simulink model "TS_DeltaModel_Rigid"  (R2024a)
settings: Solver=ode45  StartTime=0  StopTime=2  FixedStep=1e-4  EnableMultiTasking=on
PreLoadFcn:
  | warning('off','sm:sli:setup:compile:LocalSolverNotSupported')
InitFcn:
  |  SimParam.IC = SM2_InitCondConstrFnc(RawParam,IC);
model workspace (MAT data in the model file):
  op_trim1 : opcond.OperatingReport (value not decoded)
  op_trim3 : opcond.OperatingReport (value not decoded)
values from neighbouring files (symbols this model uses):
  RawParam = RobotParamGather(ParamLib)    [DeltaModelMain_v2.m]    (also in main_TimeSimulation.m; MGI.m = y)
libraries: SM2_BallJointPartsLib x6, SM2_ForeArmPartsLib x6, simulink x6, SM2_ArmPartsLib x3, SM2_MotorPartsLib x3, SM2_FramePartsLib x1, ElecDriverLib x1, SM2_ToolPartsLib x1

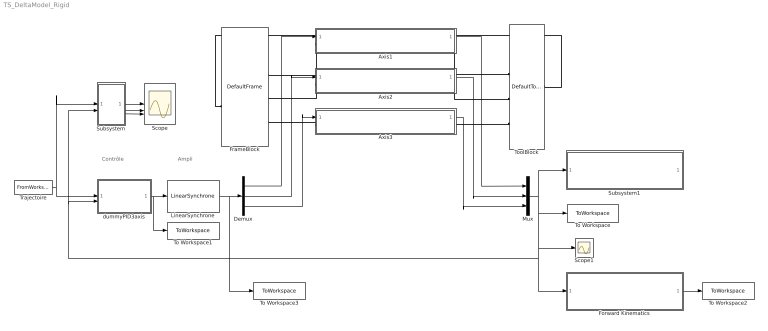
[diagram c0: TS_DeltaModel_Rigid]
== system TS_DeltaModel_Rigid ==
  note: Contrôle
  note: Ampli
  Axis1 : Subsystem  mask{AxisID=1}
      mask prompts: AxisID "Axis ID number (1,2 or 3)"
  Axis2 : Subsystem  mask{AxisID=2}
      mask prompts: AxisID "Axis ID number (1,2 or 3)"
  Axis3 : Subsystem  mask{AxisID=3}
      mask prompts: AxisID "Axis ID number (1,2 or 3)"
  Demux : Demux  Outputs=3
  Forward Kinematics : Subsystem
  FrameBlock : SM2_FramePartsLib/DefaultFrame  SystemSampleTime=-1  VariantActivationTime=update diagram  AllowFlexibleInterface=on  Latency=0  AutoFrameSizeCalculation=off
  LinearSynchrone : ElecDriverLib/LinearSynchrone  SystemSampleTime=-1  VariantControl=driverVarLinearSynchrone  VariantActivationTime=update diagram  AllowFlexibleInterface=on  Latency=0  AutoFrameSizeCalculation=off
  Mux : Mux  Inputs=3
  Scope : Scope  NumInputPorts=3
  Scope1 : Scope
  Subsystem : Subsystem
  Subsystem1 : Subsystem
  To Workspace : ToWorkspace  VariableName=angleData  SaveFormat=Timeseries  SampleTime=-1
  To Workspace1 : ToWorkspace  VariableName=controlData  SaveFormat=Timeseries  SampleTime=-1
  To Workspace2 : ToWorkspace  VariableName=endEffectorPos  SaveFormat=Structure With Time  SampleTime=-1
  To Workspace3 : ToWorkspace  VariableName=Torques  SaveFormat=Structure With Time  SampleTime=-1
  ToolBlock : SM2_ToolPartsLib/DefaultTool  SystemSampleTime=-1  VariantActivationTime=update diagram  AllowFlexibleInterface=on  Latency=0  AutoFrameSizeCalculation=off
      link override NacelleGraph: ExtrusionLength=0.005  Mass=SimParam.Tool.m
  Trajectoire : FromWorkspace  VariableName=simin  SampleTime=SimParam.Control.Te  ZeroCross=off  OutputAfterFinalValue=Holding final value
  dummyPID3axis : Subsystem  InitFcn=SimParam.Control = Control_ParamInitFnc(RawParam,3);  VariantControl=controlVarDefault
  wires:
  LinearSynchrone/1 -> To Workspace3/1, Demux/1
  Mux/1 -> Scope1/1, Forward Kinematics/1(q), Subsystem/2(y), dummyPID3axis/2(Alpha), To Workspace/1, Subsystem1/1(In1)
  dummyPID3axis/1(U) -> To Workspace1/1, LinearSynchrone/1
  Trajectoire/1 -> Subsystem/1(y_c), dummyPID3axis/1(Alpha_c)
  Demux/2 -> Axis2/1(Torque)
  Demux/3 -> Axis3/1(Torque)
  Axis1/1(Alpha) -> Mux/1
  Axis2/1(Alpha) -> Mux/2
  Axis3/1(Alpha) -> Mux/3
  Demux/1 -> Axis1/1(Torque)
  Subsystem/1(axe1) -> Scope/1
  Subsystem/2(axe2) -> Scope/2
  Subsystem/3(axe3) -> Scope/3
  Forward Kinematics/1(Out1) -> To Workspace2/1
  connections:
  Axis1/LConn1 -- FrameBlock/RConn1
  Axis2/LConn1 -- FrameBlock/RConn2
  Axis3/LConn1 -- FrameBlock/RConn3
  Axis3/RConn1 -- ToolBlock/RConn3
  Axis2/RConn1 -- ToolBlock/RConn2
  Axis1/RConn1 -- ToolBlock/RConn1
  FrameBlock/LConn1 -- ToolBlock/LConn1

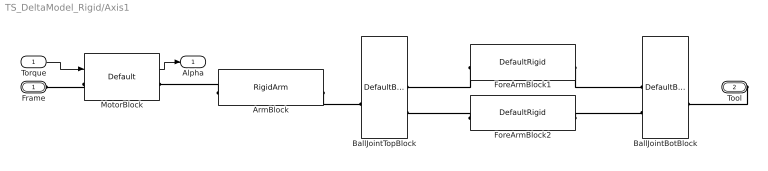
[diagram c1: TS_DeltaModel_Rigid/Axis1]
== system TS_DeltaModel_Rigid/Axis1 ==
  Torque : Inport
  ArmBlock : SM2_ArmPartsLib/RigidArm  SystemSampleTime=-1  VariantControl=armVarDefault  VariantActivationTime=update diagram  AllowFlexibleInterface=on  Latency=0  AutoFrameSizeCalculation=off
      link override ArmGraph: ExtrusionCrossSection=[5.5e-3 0; 2.75e-3 4.76e-3; -2.75e-3 4.76e-3; -5.5e-3 0; -2.75e-3 -4.76e-3; 2.75e-3 -4.76e-3; 5.5e-3 0]
  BallJointBotBlock : SM2_BallJointPartsLib/DefaultBallJointBotPair  SystemSampleTime=-1  VariantActivationTime=update diagram  AllowFlexibleInterface=on  Latency=0  AutoFrameSizeCalculation=off
  BallJointTopBlock : SM2_BallJointPartsLib/DefaultBallJointTopPair  SystemSampleTime=-1  VariantActivationTime=update diagram  AllowFlexibleInterface=on  Latency=0  AutoFrameSizeCalculation=off
  ForeArmBlock1 : SM2_ForeArmPartsLib/DefaultRigid  SystemSampleTime=-1  VariantControl=foreArmVarDefault  VariantActivationTime=update diagram  AllowFlexibleInterface=on  Latency=0  AutoFrameSizeCalculation=off
      link override ForeArmGraph: Density=SimParam.ForeArm.m  BasedOnType=Mass  Mass=SimParam.ForeArm.m  CylinderRadius=0.004025
  ForeArmBlock2 : SM2_ForeArmPartsLib/DefaultRigid  SystemSampleTime=-1  VariantControl=foreArmVarDefault  VariantActivationTime=update diagram  AllowFlexibleInterface=on  Latency=0  AutoFrameSizeCalculation=off
      link override ForeArmGraph: CylinderRadius=0.004025  BasedOnType=Mass  Mass=SimParam.ForeArm.m
  MotorBlock : SM2_MotorPartsLib/Default  SystemSampleTime=-1  VariantControl=motorVarDefault  VariantActivationTime=update diagram  AllowFlexibleInterface=on  Latency=0  AutoFrameSizeCalculation=off
  Frame : PMIOPort  Side=Left
  Tool : PMIOPort  Port=2  Side=Right
  Alpha : Outport
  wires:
  Torque/1 -> MotorBlock/1
  MotorBlock/1 -> Alpha/1
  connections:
  ArmBlock/LConn1 -- MotorBlock/RConn1
  MotorBlock/LConn1 -- Frame/RConn1
  ArmBlock/RConn1 -- BallJointTopBlock/RConn1
  Tool/RConn1 -- BallJointBotBlock/RConn1
  ForeArmBlock2/LConn1 -- BallJointTopBlock/LConn2
  ForeArmBlock1/LConn1 -- BallJointTopBlock/LConn1
  ForeArmBlock1/RConn1 -- BallJointBotBlock/LConn1
  ForeArmBlock2/RConn1 -- BallJointBotBlock/LConn2

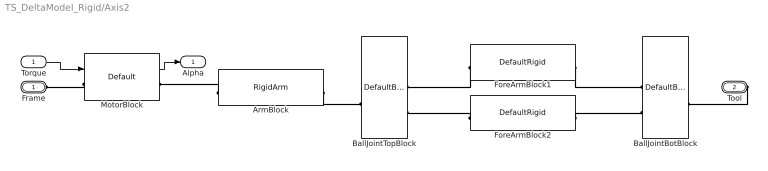
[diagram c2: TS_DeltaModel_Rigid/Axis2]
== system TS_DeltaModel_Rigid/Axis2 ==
  Torque : Inport
  ArmBlock : SM2_ArmPartsLib/RigidArm  SystemSampleTime=-1  VariantControl=armVarDefault  VariantActivationTime=update diagram  AllowFlexibleInterface=on  Latency=0  AutoFrameSizeCalculation=off
  BallJointBotBlock : SM2_BallJointPartsLib/DefaultBallJointBotPair  SystemSampleTime=-1  VariantActivationTime=update diagram  AllowFlexibleInterface=on  Latency=0  AutoFrameSizeCalculation=off
  BallJointTopBlock : SM2_BallJointPartsLib/DefaultBallJointTopPair  SystemSampleTime=-1  VariantActivationTime=update diagram  AllowFlexibleInterface=on  Latency=0  AutoFrameSizeCalculation=off
  ForeArmBlock1 : SM2_ForeArmPartsLib/DefaultRigid  SystemSampleTime=-1  VariantControl=foreArmVarDefault  VariantActivationTime=update diagram  AllowFlexibleInterface=on  Latency=0  AutoFrameSizeCalculation=off
      link override ForeArmGraph: CylinderRadius=0.004025  BasedOnType=Mass  Mass=SimParam.ForeArm.m
  ForeArmBlock2 : SM2_ForeArmPartsLib/DefaultRigid  SystemSampleTime=-1  VariantControl=foreArmVarDefault  VariantActivationTime=update diagram  AllowFlexibleInterface=on  Latency=0  AutoFrameSizeCalculation=off
      link override ForeArmGraph: CylinderRadius=0.004025  BasedOnType=Mass  Mass=SimParam.ForeArm.m
  MotorBlock : SM2_MotorPartsLib/Default  SystemSampleTime=-1  VariantControl=motorVarDefault  VariantActivationTime=update diagram  AllowFlexibleInterface=on  Latency=0  AutoFrameSizeCalculation=off
  Frame : PMIOPort  Side=Left
  Tool : PMIOPort  Port=2  Side=Right
  Alpha : Outport
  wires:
  Torque/1 -> MotorBlock/1
  MotorBlock/1 -> Alpha/1
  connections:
  ArmBlock/LConn1 -- MotorBlock/RConn1
  MotorBlock/LConn1 -- Frame/RConn1
  ArmBlock/RConn1 -- BallJointTopBlock/RConn1
  Tool/RConn1 -- BallJointBotBlock/RConn1
  ForeArmBlock2/LConn1 -- BallJointTopBlock/LConn2
  ForeArmBlock1/LConn1 -- BallJointTopBlock/LConn1
  ForeArmBlock1/RConn1 -- BallJointBotBlock/LConn1
  ForeArmBlock2/RConn1 -- BallJointBotBlock/LConn2

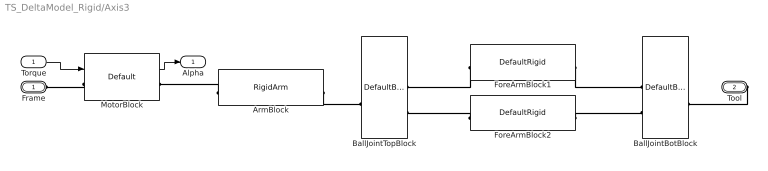
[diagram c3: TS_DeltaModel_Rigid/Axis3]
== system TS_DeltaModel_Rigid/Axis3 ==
  Torque : Inport
  ArmBlock : SM2_ArmPartsLib/RigidArm  SystemSampleTime=-1  VariantControl=armVarDefault  VariantActivationTime=update diagram  AllowFlexibleInterface=on  Latency=0  AutoFrameSizeCalculation=off
  BallJointBotBlock : SM2_BallJointPartsLib/DefaultBallJointBotPair  SystemSampleTime=-1  VariantActivationTime=update diagram  AllowFlexibleInterface=on  Latency=0  AutoFrameSizeCalculation=off
  BallJointTopBlock : SM2_BallJointPartsLib/DefaultBallJointTopPair  SystemSampleTime=-1  VariantActivationTime=update diagram  AllowFlexibleInterface=on  Latency=0  AutoFrameSizeCalculation=off
  ForeArmBlock1 : SM2_ForeArmPartsLib/DefaultRigid  SystemSampleTime=-1  VariantControl=foreArmVarDefault  VariantActivationTime=update diagram  AllowFlexibleInterface=on  Latency=0  AutoFrameSizeCalculation=off
      link override ForeArmGraph: CylinderRadius=0.004025  BasedOnType=Mass  Mass=SimParam.ForeArm.m
  ForeArmBlock2 : SM2_ForeArmPartsLib/DefaultRigid  SystemSampleTime=-1  VariantControl=foreArmVarDefault  VariantActivationTime=update diagram  AllowFlexibleInterface=on  Latency=0  AutoFrameSizeCalculation=off
      link override ForeArmGraph: CylinderRadius=0.004025  BasedOnType=Mass  Mass=SimParam.ForeArm.m
  MotorBlock : SM2_MotorPartsLib/Default  SystemSampleTime=-1  VariantControl=motorVarDefault  VariantActivationTime=update diagram  AllowFlexibleInterface=on  Latency=0  AutoFrameSizeCalculation=off
  Frame : PMIOPort  Side=Left
  Tool : PMIOPort  Port=2  Side=Right
  Alpha : Outport
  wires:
  Torque/1 -> MotorBlock/1
  MotorBlock/1 -> Alpha/1
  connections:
  ArmBlock/LConn1 -- MotorBlock/RConn1
  MotorBlock/LConn1 -- Frame/RConn1
  ArmBlock/RConn1 -- BallJointTopBlock/RConn1
  Tool/RConn1 -- BallJointBotBlock/RConn1
  ForeArmBlock2/LConn1 -- BallJointTopBlock/LConn2
  ForeArmBlock1/LConn1 -- BallJointTopBlock/LConn1
  ForeArmBlock1/RConn1 -- BallJointBotBlock/LConn1
  ForeArmBlock2/RConn1 -- BallJointBotBlock/LConn2

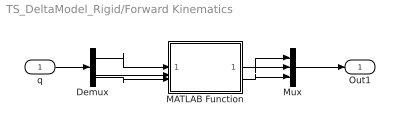
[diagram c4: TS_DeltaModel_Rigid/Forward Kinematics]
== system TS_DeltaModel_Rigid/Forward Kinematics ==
  q : Inport
  Demux : Demux  Outputs=3
  MATLAB Function : MATLAB Function  TreatAsAtomicUnit=on
  Mux : Mux  Inputs=3
  Out1 : Outport
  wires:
  q/1 -> Demux/1
  Demux/1 -> MATLAB Function/1(q1)
  Demux/2 -> MATLAB Function/2(q2)
  Demux/3 -> MATLAB Function/3(q3)
  MATLAB Function/1(x) -> Mux/1
  MATLAB Function/2(y) -> Mux/2
  MATLAB Function/3(z) -> Mux/3
  Mux/1 -> Out1/1

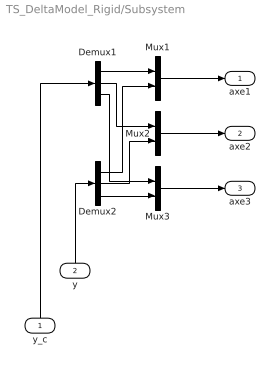
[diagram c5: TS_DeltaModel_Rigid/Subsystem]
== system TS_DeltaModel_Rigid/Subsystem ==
  y_c : Inport
  y : Inport  Port=2
  Demux1 : Demux  Outputs=3
  Demux2 : Demux  Outputs=3
  Mux1 : Mux  Inputs=2
  Mux2 : Mux  Inputs=2
  Mux3 : Mux  Inputs=2
  axe1 : Outport
  axe2 : Outport  Port=2
  axe3 : Outport  Port=3
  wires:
  Demux1/3 -> Mux3/1
  Demux1/1 -> Mux1/1
  Demux2/1 -> Mux1/2
  Mux1/1 -> axe1/1
  Demux1/2 -> Mux2/1
  Demux2/2 -> Mux2/2
  y/1 -> Demux2/1
  Demux2/3 -> Mux3/2
  Mux3/1 -> axe3/1
  y_c/1 -> Demux1/1
  Mux2/1 -> axe2/1

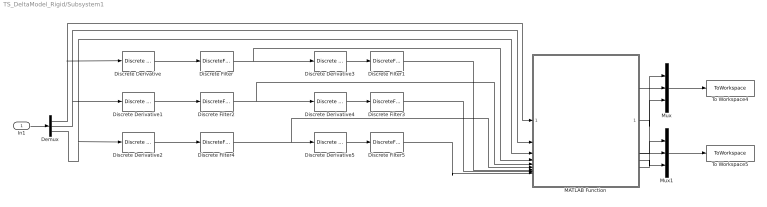
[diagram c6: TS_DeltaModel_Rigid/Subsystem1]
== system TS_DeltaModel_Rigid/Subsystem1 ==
  In1 : Inport
  Demux : Demux  Outputs=3
  Discrete Derivative{,1..5} (6 alike) : simulink/Discrete/Discrete Derivative  gainval=1.0  ICPrevScaledInput=0.0  OutMin=[]  OutMax=[]  OutDataType=fixdt(1, 16)  OutScaling=2^-10  DoSatur=off
  Discrete Filter{,1..5} (6 alike) : DiscreteFilter  Denominator=[-(1-0.3)]
  MATLAB Function : MATLAB Function  TreatAsAtomicUnit=on
  Mux : Mux  Inputs=3
  Mux1 : Mux  Inputs=3
  To Workspace4 : ToWorkspace  VariableName=endEffectorVel  SaveFormat=Structure With Time  SampleTime=-1
  To Workspace5 : ToWorkspace  VariableName=endEffectorAcc  SaveFormat=Structure With Time  SampleTime=-1
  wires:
  In1/1 -> Demux/1
  Demux/1 -> Discrete Derivative/1, MATLAB Function/1(q1)
  Demux/2 -> Discrete Derivative1/1, MATLAB Function/2(q2)
  Demux/3 -> Discrete Derivative2/1, MATLAB Function/3(q3)
  Discrete Derivative/1 -> Discrete Filter/1
  Discrete Derivative1/1 -> Discrete Filter2/1
  Discrete Derivative2/1 -> Discrete Filter4/1
  Discrete Derivative5/1 -> Discrete Filter5/1
  Discrete Derivative4/1 -> Discrete Filter3/1
  Discrete Derivative3/1 -> Discrete Filter1/1
  MATLAB Function/2(endEffectorVelY) -> Mux/2
  MATLAB Function/1(endEffectorVelX) -> Mux/1
  MATLAB Function/3(endEffectorVelZ) -> Mux/3
  MATLAB Function/5(endEffectorAccY) -> Mux1/2
  MATLAB Function/4(endEffectorAccX) -> Mux1/1
  MATLAB Function/6(endEffectorAccZ) -> Mux1/3
  Mux/1 -> To Workspace4/1
  Mux1/1 -> To Workspace5/1
  Discrete Filter/1 -> MATLAB Function/4(q1_dot), Discrete Derivative3/1
  Discrete Filter1/1 -> MATLAB Function/7(q1_ddot)
  Discrete Filter2/1 -> Discrete Derivative4/1, MATLAB Function/5(q2_dot)
  Discrete Filter3/1 -> MATLAB Function/8(q2_ddot)
  Discrete Filter4/1 -> MATLAB Function/6(q3_dot), Discrete Derivative5/1
  Discrete Filter5/1 -> MATLAB Function/9(q3_ddot)

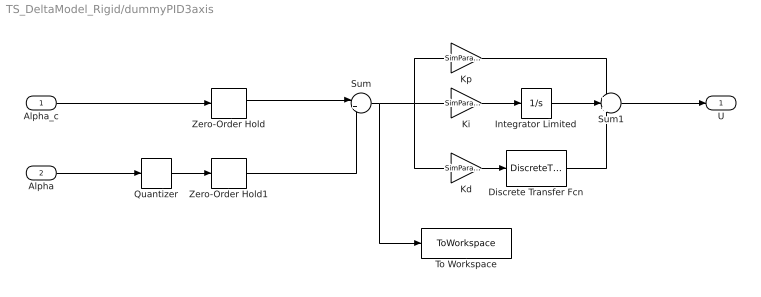
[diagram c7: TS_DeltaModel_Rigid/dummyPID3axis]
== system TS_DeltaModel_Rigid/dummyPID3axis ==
  Alpha_c : Inport
  Alpha : Inport  Port=2
  Discrete Transfer Fcn : DiscreteTransferFcn  Numerator=[1 0 -1]  Denominator=[2 0 0]
  Integrator Limited : Integrator  LimitOutput=on  UpperSaturationLimit=3000  LowerSaturationLimit=-3000
  Kd : Gain  Gain=SimParam.Control.Kd/SimParam.Control.Te
  Ki : Gain  Gain=SimParam.Control.Ki*SimParam.Control.Te
  Kp : Gain  Gain=SimParam.Control.Kp
  Quantizer : Quantizer  QuantizationInterval=2*pi/(4500*4*25)
  Sum : Sum  Inputs=|+-
  Sum1 : Sum  Inputs=+++
  To Workspace : ToWorkspace  VariableName=errorData  SaveFormat=Timeseries  SampleTime=-1
  Zero-Order Hold : ZeroOrderHold  SampleTime=SimParam.Control.Te
  Zero-Order Hold1 : ZeroOrderHold  SampleTime=SimParam.Control.Te
  U : Outport
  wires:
  Sum1/1 -> U/1
  Alpha/1 -> Quantizer/1
  Alpha_c/1 -> Zero-Order Hold/1
  Zero-Order Hold1/1 -> Sum/2
  Sum/1 -> To Workspace/1, Kd/1, Kp/1, Ki/1
  Integrator Limited/1 -> Sum1/2
  Ki/1 -> Integrator Limited/1
  Kp/1 -> Sum1/1
  Discrete Transfer Fcn/1 -> Sum1/3
  Quantizer/1 -> Zero-Order Hold1/1
  Zero-Order Hold/1 -> Sum/1
  Kd/1 -> Discrete Transfer Fcn/1

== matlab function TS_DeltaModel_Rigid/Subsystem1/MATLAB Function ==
function [endEffectorVelX, endEffectorVelY, endEffectorVelZ, endEffectorAccX, endEffectorAccY, endEffectorAccZ] = calcVelAcc(q1, q2, q3, q1_dot, q2_dot, q3_dot, q1_ddot, q2_ddot, q3_ddot)
    % Create vectors with explicit dimensions
    q = zeros(3,1);
    q(1) = q1; q(2) = q2; q(3) = q3;
    
    q_dot = zeros(3,1);
    q_dot(1) = q1_dot; q_dot(2) = q2_dot; q_dot(3) = q3_dot;
    
    q_ddot = zeros(3,1);
    q_ddot(1) = q1_ddot; q_ddot(2) = q2_ddot; q_ddot(3) = q3_ddot;
    
    % Calculate velocity and acceleration
    [vel, acc] = deltaVelAcc(q, q_dot, q_ddot);
    
    % Output scalar components
    endEffectorVelX = vel(1);
    endEffectorVelY = vel(2);
    endEffectorVelZ = vel(3);
    
    endEffectorAccX = acc(1);
    endEffectorAccY = acc(2);
    endEffectorAccZ = acc(3);
end

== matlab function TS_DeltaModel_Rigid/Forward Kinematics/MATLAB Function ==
function [x, y, z] = Position(q1, q2, q3)

    [x, y, z] = deltaForwardKinematics(q1, q2, q3);

end
